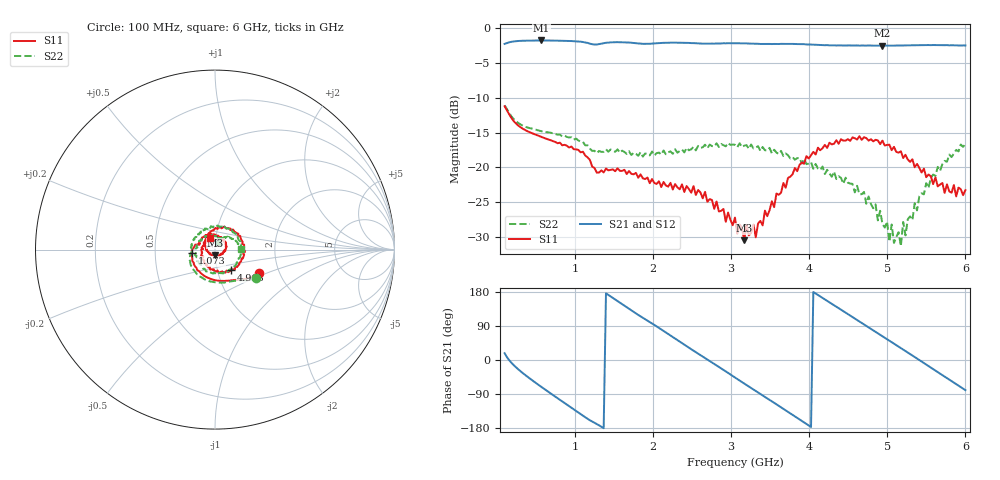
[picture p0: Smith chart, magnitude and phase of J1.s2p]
!Agilent Technologies,E8364B,MY43040379,A.07.50.67
!Agilent E8364B: A.07.50.67
!Date: Tuesday, March 24, 2026 11:03:29
!Correction: S11(Full 2 Port(1,2))
!S21(Full 2 Port(1,2))
!S12(Full 2 Port(1,2))
!S22(Full 2 Port(1,2))
!S2P File: Measurements: S11, S21, S12, S22:
# Hz S  dB  R 50
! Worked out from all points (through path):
!   201 points, 100 MHz to 6 GHz, reference 50 ohm
!   highest |S21| = -1.73 dB at 572 MHz (marker M1); lowest = -2.5 dB at 4.938 GHz (marker M2)
!   group delay of S21, straight-line fit = 373 ps
!   lowest |S11| = -30.5 dB at 3.168 GHz (marker M3), VSWR 1.06, Z = 50.1 - j3 ohm
!   |S11| at or under -10 dB: start of sweep to end of sweep
!   |S22| runs from -31.3 to -11.1 dB; largest |S21 - S12| = 0.0043
!   S11 on the Smith chart (normalised r, x): 100 MHz: 1.57, -0.44; 1.073 GHz: 0.77, -0.03; 4.968 GHz: 1.17, -0.27; 6 GHz: 0.94, +0.12
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1e8  -11.20 -28.1  -2.23 18.0  -2.23 17.8  -11.06 -34.4
3.065e8  -14.24 -62.1  -1.79 -30.2  -1.80 -30.4  -13.83 -59.3
5.72e8  -15.61 -97.4  -1.73 -71.2  -1.75 -71.5  -14.80 -89.3
8.08e8  -16.44 -131.7  -1.78 -105.1  -1.79 -105.4  -15.27 -120.6
1.0735e9  -17.83 -171.5  -1.91 -142.7  -1.92 -142.9  -16.29 -153.9
1.103e9  -17.73 -177.7  -1.95 -146.9  -1.97 -147.2  -16.32 -159.6
1.5455e9  -20.12 137.7  -1.98 155.4  -1.99 155.1  -17.40 158.0
2.0765e9  -21.99 78.0  -2.11 84.7  -2.12 84.4  -17.86 103.5
2.578e9  -23.24 28.0  -2.15 16.7  -2.17 16.4  -16.89 50.2
3.05e9  -27.21 -57.9  -2.12 -46.2  -2.14 -46.4  -16.74 -18.0
3.168e9  -30.46 -87.0  -2.16 -62.2  -2.17 -62.3  -16.87 -32.7
3.5515e9  -25.71 160.0  -2.24 -113.1  -2.25 -113.3  -17.44 -94.7
4.053e9  -17.76 73.9  -2.33 179.4  -2.34 179.3  -20.19 172.9
4.525e9  -16.18 11.9  -2.45 117.3  -2.47 117.0  -22.32 97.1
4.938e9  -16.14 -44.6  -2.49 62.6  -2.50 62.6  -28.14 38.8
4.9675e9  -16.84 -50.5  -2.48 58.8  -2.49 58.6  -28.64 52.8
5.0265e9  -16.72 -59.6  -2.47 50.9  -2.48 50.9  -30.67 46.9
5.056e9  -17.51 -60.8  -2.47 47.1  -2.49 46.8  -28.20 54.1
5.174e9  -17.68 -81.0  -2.46 31.4  -2.46 31.3  -31.32 69.3
5.2035e9  -18.64 -83.0  -2.45 27.5  -2.46 27.3  -27.83 66.8
5.4985e9  -21.40 -134.6  -2.40 -12.0  -2.42 -12.2  -22.25 60.4
6e9  -23.26 115.7  -2.45 -79.5  -2.47 -79.6  -16.64 2.1
